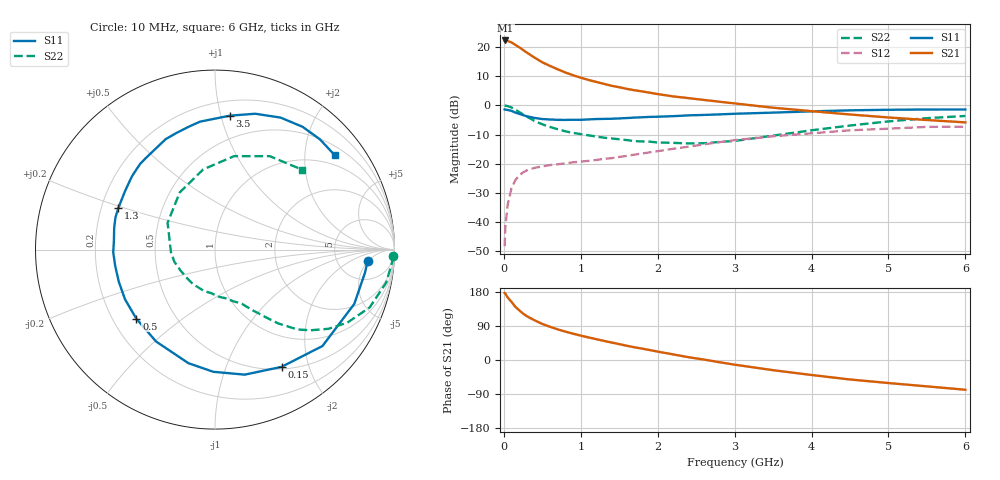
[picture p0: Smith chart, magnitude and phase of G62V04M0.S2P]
! SIEMENS Small Signal Semiconductors
! BFG193
! Si NPN RF Bipolar Junction Transistor in SOT223
! VCE = 2 V  IC = 4 mA
! Common Emitter S-Parameters:  August  1996
# GHz  S  MA  R  50
!  f  S11  S21  S12  S22
! GHz  MAG  ANG  MAG  ANG  MAG  ANG  MAG  ANG
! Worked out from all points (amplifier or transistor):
!   36 points, 10 MHz to 6 GHz, reference 50 ohm
!   highest |S21| = 22.2 dB at 20 MHz (marker M1)
!   |S21| within 3 dB of that: start of sweep to 236.1 MHz
!   unconditionally stable (mu >= 1): 1.184 GHz to 2.712 GHz
!   at 250 MHz: K = 0.29, MSG = 20.9 dB, |S12| = -22.9 dB
!   at 1.4 GHz: K = 1.10, MAG = 10.5 dB, |S12| = -18.1 dB
!   at 6 GHz: K = 0.93, MSG = 0.7 dB, |S12| = -7.3 dB
!   S11 on the Smith chart (normalised r, x): 10 MHz: 10, -5; 150 MHz: 0.53, -1.59; 500 MHz: 0.30, -0.35; 1.3 GHz: 0.27, +0.19; 3.5 GHz: 0.31, +1.07; 6 GHz: 0.72, +2.72
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0.01  0.8527 -4.3  12.84 177.0  0.0039 90.3  0.9933 -2.2
0.02  0.8456 -8.7  12.88 174.9  0.0083 86.3  0.9883 -4.4
0.05  0.8329 -21.3  12.64 165.0  0.02 77.8  0.9715 -10.9
0.1  0.8044 -41.9  11.89 153.2  0.0384 69.0  0.9199 -20.5
0.15  0.7512 -60.4  10.83 140.3  0.0526 59.5  0.8423 -28.9
0.2  0.7162 -76.6  9.849 131.2  0.063 53.5  0.7709 -34.9
0.25  0.6808 -90.8  8.853 122.5  0.0713 47.5  0.6978 -40.1
0.3  0.6499 -103.2  7.97 115.5  0.0774 43.8  0.6395 -44.1
0.4  0.6082 -122.7  6.541 104.7  0.0853 38.2  0.5405 -49.5
0.5  0.5833 -138.7  5.451 95.1  0.0904 34.3  0.4734 -53.0
0.6  0.5727 -151.1  4.721 87.6  0.0951 32.8  0.4267 -55.9
0.7  0.5651 -161.7  4.135 80.8  0.098 31.7  0.3904 -58.9
0.9  0.5672 -178.5  3.273 69.4  0.106 30.9  0.3378 -63.5
1.1  0.5744 168.0  2.719 59.6  0.1123 31.3  0.307 -70.1
1.3  0.5864 156.8  2.33 50.5  0.1214 32.0  0.2798 -76.6
1.7  0.6173 138.4  1.811 33.5  0.1434 32.4  0.2443 -94.1
2.2  0.6525 120.4  1.423 14.8  0.1806 28.8  0.2284 -122.4
2.8  0.6999 102.1  1.154 -5.8  0.2346 20.8  0.2363 -163.2
3.5  0.7508 83.7  0.911 -26.9  0.2956 6.0  0.3035 150.5
4.5  0.8212 63.6  0.698 -51.4  0.374 -14.6  0.4515 98.4
5.5  0.8481 46.4  0.561 -69.6  0.428 -40.2  0.6035 59.6
6  0.8494 38.2  0.511 -78.5  0.4316 -54.5  0.6579 42.7
